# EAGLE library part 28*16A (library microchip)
CMOS EPROM 16 K (2 K x 8) Source: ww1.microchip.com/downloads/en/DeviceDoc/11125J.pdf
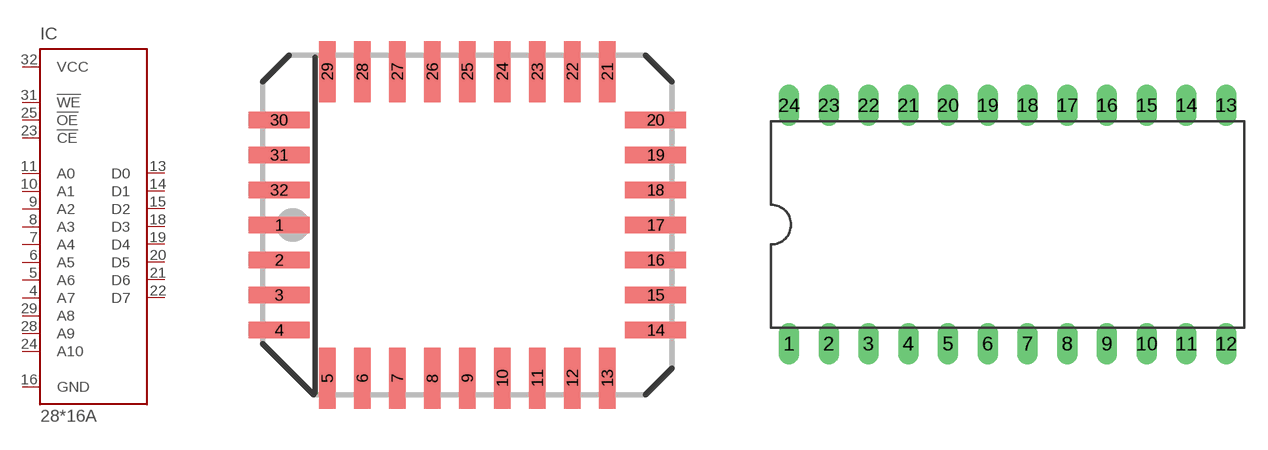
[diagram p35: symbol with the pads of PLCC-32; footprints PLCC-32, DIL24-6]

Designator prefix IC

## 28C16AL (MPN: CAT28C16AGI-12; OC_FARNELL: 1718288; OC_NEWARK: 06R0639)  [PLCC-32]
4  A7  in
5  A6  in
6  A5  in
7  A4  in
8  A3  in
9  A2  in
10  A1  in
11  A0  in
13  D0  hiz
14  D1  hiz
15  D2  hiz
16  GND  pwr
18  D3  hiz
19  D4  hiz
20  D5  hiz
21  D6  hiz
22  D7  hiz
23  !CE  in
24  A10  in
25  !OE  in
28  A9  in
29  A8  in
31  !WE  in
32  VCC  pwr

## 28C16AP (MPN: CAT28C16ALI-12; OC_FARNELL: 1718292; OC_NEWARK: 06R0648)  [DIL24-6]
1  A7  in
2  A6  in
3  A5  in
4  A4  in
5  A3  in
6  A2  in
7  A1  in
8  A0  in
9  D0  hiz
10  D1  hiz
11  D2  hiz
12  GND  pwr
13  D3  hiz
14  D4  hiz
15  D5  hiz
16  D6  hiz
17  D7  hiz
18  !CE  in
19  A10  in
20  !OE  in
21  !WE  in
22  A9  in
23  A8  in
24  VCC  pwr

## 28C16ATS (OC_FARNELL: unknown; OC_NEWARK: unknown)  [TSOP28]
1  !OE  in
3  A9  in
4  A8  in
6  !WE  in
7  VCC  pwr
10  A7  in
11  A6  in
12  A5  in
13  A4  in
14  A3  in
15  A2  in
16  A1  in
17  A0  in
18  D0  hiz
19  D1  hiz
20  D2  hiz
21  GND  pwr
22  D3  hiz
23  D4  hiz
24  D5  hiz
25  D6  hiz
26  D7  hiz
27  !CE  in
28  A10  in

## 28C16AVS (OC_FARNELL: 1718287; OC_NEWARK: unknown)  [VSOP28-8X13]
3  A7  in
4  A6  in
5  A5  in
6  A4  in
7  A3  in
8  A2  in
9  A1  in
10  A0  in
11  D0  hiz
12  D1  hiz
13  D2  hiz
14  GND  pwr
15  D3  hiz
16  D4  hiz
17  D5  hiz
18  D6  hiz
19  D7  hiz
20  !CE  in
21  A10  in
22  !OE  in
24  A9  in
25  A8  in
27  !WE  in
28  VCC  pwr

## Footprint PLCC-32 (pad centres in mm)
PLASTIC LEADED CHIP CARRIER rectangle, package type L
smd 2.2 x 0.6: 1 -6.83,0; 2 -6.83,-1.27; 3 -6.83,-2.54; 4 -6.83,-3.81; 14 6.83,-3.81; 15 6.83,-2.54; 16 6.83,-1.27; 17 6.83,0; 18 6.83,1.27; 19 6.83,2.54; 20 6.83,3.81; 30 -6.83,3.81; 31 -6.83,2.54; 32 -6.83,1.27
smd 0.6 x 2.2: 5 -5.08,-5.56; 6 -3.81,-5.56; 7 -2.54,-5.56; 8 -1.27,-5.56; 9 0,-5.56; 10 1.27,-5.56; 11 2.54,-5.56; 12 3.81,-5.56; 13 5.08,-5.56; 21 5.08,5.56; 22 3.81,5.56; 23 2.54,5.56; 24 1.27,5.56; 25 0,5.56; 26 -1.27,5.56; 27 -2.54,5.56; 28 -3.81,5.56; 29 -5.08,5.56

## Footprint DIL24-6 (pad centres in mm)
Dual In Line package type P
drill 0.813 long: 1 -13.97,-7.62; 2 -11.43,-7.62; 3 -8.89,-7.62; 4 -6.35,-7.62; 5 -3.81,-7.62; 6 -1.27,-7.62; 7 1.27,-7.62; 8 3.81,-7.62; 9 6.35,-7.62; 10 8.89,-7.62; 11 11.43,-7.62; 12 13.97,-7.62; 13 13.97,7.62; 14 11.43,7.62; 15 8.89,7.62; 16 6.35,7.62; 17 3.81,7.62; 18 1.27,7.62; 19 -1.27,7.62; 20 -3.81,7.62; 21 -6.35,7.62; 22 -8.89,7.62; 23 -11.43,7.62; 24 -13.97,7.62

## Footprint TSOP28 (pad centres in mm)
Thin Small Outline Package Gull Wing type I, package type TS
smd 0.3 x 1: 1 -3.75,-9.7; 2 -3.25,-9.7; 3 -2.75,-9.7; 4 -2.25,-9.7; 5 -1.75,-9.7; 6 -1.25,-9.7; 7 -0.75,-9.7; 8 0.75,-9.7; 9 1.25,-9.7; 10 1.75,-9.7; 11 2.25,-9.7; 12 2.75,-9.7; 13 3.25,-9.7; 14 3.75,-9.7; 15 3.75,9.7; 16 3.25,9.7; 17 2.75,9.7; 18 2.25,9.7; 19 1.75,9.7; 20 1.25,9.7; 21 0.75,9.7; 22 -0.75,9.7; 23 -1.25,9.7; 24 -1.75,9.7; 25 -2.25,9.7; 26 -2.75,9.7; 27 -3.25,9.7; 28 -3.75,9.7

## Footprint VSOP28-8X13 (pad centres in mm)
Very Small Outline Package 8 x 13.4 mm, package type VS
smd 0.3 x 1.1: 1 0.275,-6.45; 2 0.825,-6.45; 3 1.375,-6.45; 4 1.925,-6.45; 5 2.475,-6.45; 6 3.025,-6.45; 7 3.575,-6.45; 8 3.575,6.45; 9 3.025,6.45; 10 2.475,6.45; 11 1.925,6.45; 12 1.375,6.45; 13 0.825,6.45; 14 0.275,6.45; 15 -0.275,6.45; 16 -0.825,6.45; 17 -1.375,6.45; 18 -1.925,6.45; 19 -2.475,6.45; 20 -3.025,6.45; 21 -3.575,6.45; 22 -3.575,-6.45; 23 -3.025,-6.45; 24 -2.475,-6.45; 25 -1.925,-6.45; 26 -1.375,-6.45; 27 -0.825,-6.45; 28 -0.275,-6.45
